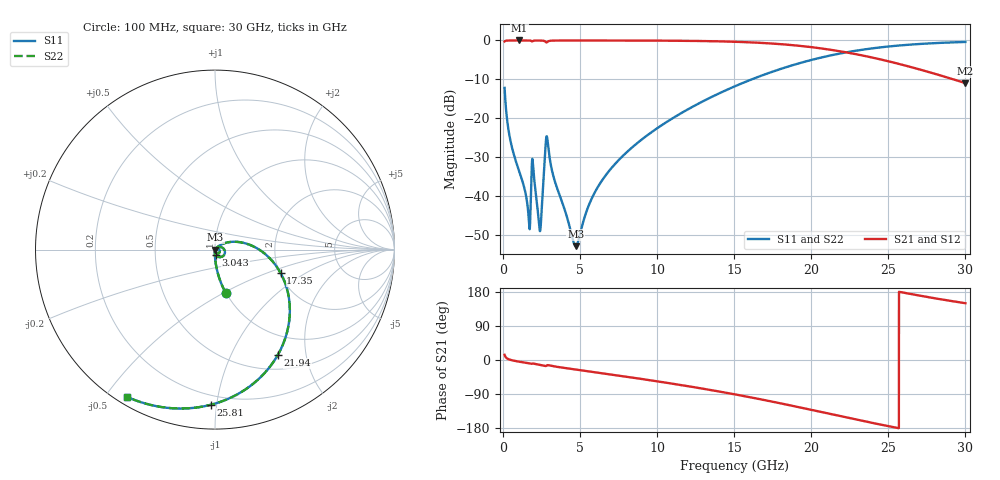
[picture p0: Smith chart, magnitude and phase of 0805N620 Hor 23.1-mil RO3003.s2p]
# GHz S MA R 50
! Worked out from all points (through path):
!   3201 points, 100 MHz to 30 GHz, reference 50 ohm
!   highest |S21| = -0.01 dB at 1.053 GHz (marker M1); lowest = -11.0 dB at 30 GHz (marker M2)
!   group delay of S21, straight-line fit = 20.3 ps
!   lowest |S11| = -52.8 dB at 4.716 GHz (marker M3), VSWR 1.00, Z = 50.2 - j0.0952 ohm
!   |S11| at or under -10 dB: start of sweep to 16.13 GHz
!   |S22| runs from -52.8 to -0.4 dB; largest |S21 - S12| = 0
!   S11 on the Smith chart (normalised r, x): 100 MHz: 1.00, -0.51; 3.043 GHz: 1.01, -0.06; 17.35 GHz: 2.02, -0.63; 21.94 GHz: 0.69, -1.53; 25.81 GHz: 0.14, -0.96; 30 GHz: 0.03, -0.57
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0.1  0.2463 -76.2  0.9689 13.7  0.9689 13.7  0.2463 -76.2
0.4644063  0.05346 -88.9  0.998 0.6  0.998 0.6  0.05346 -88.9
1.053063  0.02075 -92.2  0.9989 -4.5  0.9989 -4.5  0.02075 -92.2
1.651063  0.005624 -76.8  0.9978 -8.6  0.9978 -8.6  0.005624 -76.8
1.978094  0.0208 -72.0  0.9901 -9.6  0.9901 -9.6  0.0208 -72.0
2.370531  0.003717 -39.4  0.9966 -12.6  0.9966 -12.6  0.003717 -39.4
2.492  0.005985 23.7  0.9951 -13.6  0.9951 -13.6  0.005985 23.7
2.791  0.05408 -4.5  0.9468 -15.6  0.9468 -15.6  0.05408 -4.5
2.903125  0.04862 -59.6  0.9655 -13.6  0.9655 -13.6  0.04862 -59.6
3.043281  0.02937 -82.3  0.9883 -14.7  0.9883 -14.7  0.02937 -82.3
4.715813  0.002295 -24.4  0.9975 -25.1  0.9975 -25.1  0.002295 -24.4
5.089563  0.003907 26.8  0.9975 -27.3  0.9975 -27.3  0.003907 26.8
5.743625  0.009286 44.4  0.9974 -31.0  0.9974 -31.0  0.009286 44.4
6.706031  0.01915 46.0  0.9971 -36.5  0.9971 -36.5  0.01915 46.0
10.06978  0.07636 30.9  0.9935 -56.7  0.9935 -56.7  0.07636 30.9
15.05  0.2584 -1.8  0.9607 -90.7  0.9607 -90.7  0.2584 -1.8
17.34856  0.3888 -19.7  0.915 -108.9  0.915 -108.9  0.3888 -19.7
20.03956  0.5639 -42.6  0.8183 -131.9  0.8183 -131.9  0.5639 -42.6
21.93634  0.6835 -59.2  0.7216 -148.6  0.7216 -148.6  0.6835 -59.2
25.01978  0.8361 -85.2  0.539 -174.7  0.539 -174.7  0.8361 -85.2
25.814  0.8647 -91.5  0.4924 179.0  0.4924 179.0  0.8647 -91.5
30  0.9554 -120.7  0.2834 149.8  0.2834 149.8  0.9554 -120.7
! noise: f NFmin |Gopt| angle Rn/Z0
0.1  0.0004062  0.8525  0.724  0.0005875
3.417  0.00848  0.7708  18.32  0.007354
6.743  0.009836  0.6443  35.54  0.00477
10.06  0.01354  0.6278  51.78  0.005586
13.39  0.0178  0.6326  66.99  0.006473
16.7  0.02295  0.6511  81.14  0.00745
20.03  0.02962  0.6805  94.51  0.008613
23.35  0.03872  0.7195  107.3  0.01007
26.67  0.05204  0.7667  120  0.01195
30  0.07292  0.819  132.7  0.01427
